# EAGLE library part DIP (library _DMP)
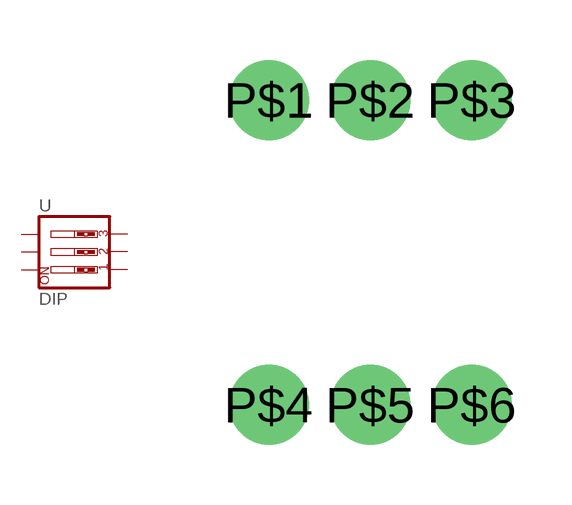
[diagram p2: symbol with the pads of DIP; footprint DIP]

Designator prefix -

## DIP  [DIP]
P$1  1  pas
P$2  2  pas
P$3  3  pas
P$4  4  pas
P$5  5  pas
P$6  6  pas

## Footprint DIP (pad centres in mm)
drill 1.1 pad 2: P$1 0,0; P$2 2.54,0; P$3 5.08,0; P$4 0,-7.62; P$5 2.54,-7.62; P$6 5.08,-7.62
